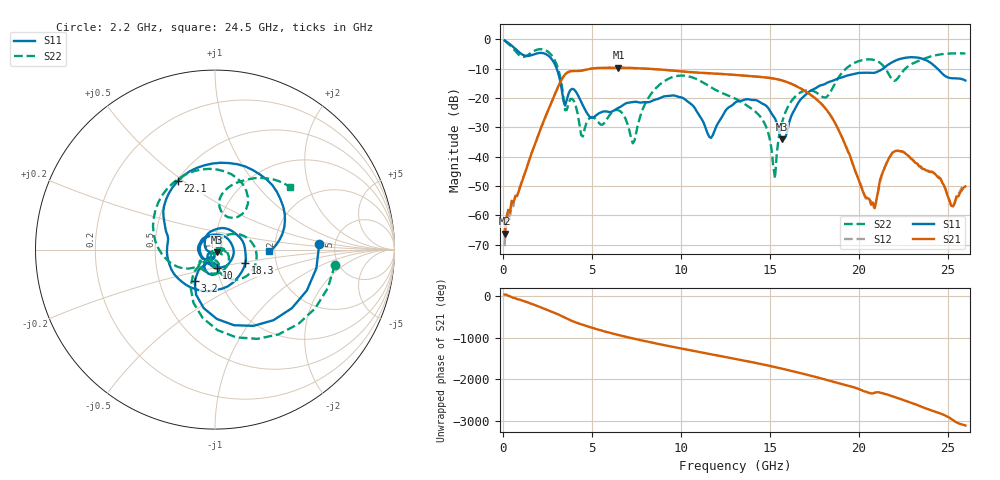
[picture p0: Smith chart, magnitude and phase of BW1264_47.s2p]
!Keysight Technologies,N5245B,MY57181159,A.13.60.06
!Date: Friday, December 18, 2020 23:54:32
!Correction: S11(Full 2 Port(1,2))
!S21(Full 2 Port(1,2))
!S12(Full 2 Port(1,2))
!S22(Full 2 Port(1,2))
!S2P File: Measurements: S11, S21, S12, S22:
# Hz S  dB  R 50
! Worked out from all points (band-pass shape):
!   260 points, 100 MHz to 26 GHz, reference 50 ohm
!   highest |S21| = -9.73 dB at 6.5 GHz (marker M1); lowest = -66.2 dB at 100 MHz (marker M2)
!   |S21| within 3 dB of the highest: 3.411 GHz to 14.2 GHz (10.79 GHz wide, 123 % of centre)
!   lowest |S11| = -34.1 dB at 15.7 GHz (marker M3), VSWR 1.04, Z = 51.2 - j1.63 ohm
!   |S11| at or under -10 dB: 3.025 GHz to 21.38 GHz (18.36 GHz wide, 150 % of centre); 24.42 GHz to end of sweep
!   |S22| runs from -47.5 to -0.5 dB; largest |S21 - S12| = 0.00049
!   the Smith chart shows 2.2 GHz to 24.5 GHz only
!   S11 on the Smith chart (normalised r, x): 2.2 GHz: 3.74, +0.38; 3.2 GHz: 0.75, -0.28; 10 GHz: 1.00, -0.21; 18.3 GHz: 1.39, -0.21; 22.1 GHz: 0.51, +0.48; 24.5 GHz: 1.85, -0.04
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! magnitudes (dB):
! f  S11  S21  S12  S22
! 100 MHz  -0.4  -66.2  -70.5  -0.5
! 300 MHz  -1.3  -58.2  -58.2  -1.5
! 2.2 GHz  -4.7  -29.4  -29.4  -3.4
! 3.2 GHz  -13.6  -15.0  -15.0  -12.1
! 4.5 GHz  -22.6  -10.6  -10.6  -33.1
! 6.5 GHz  -23.4  -9.7  -9.7  -24.2
! 7.3 GHz  -21.5  -9.8  -9.8  -35.5
! 8.8 GHz  -20.2  -10.3  -10.3  -15.6
! 10 GHz  -19.8  -11.0  -11.0  -12.4
! 11.7 GHz  -33.7  -11.7  -11.7  -16.4
! 13.1 GHz  -21.4  -12.2  -12.2  -20.3
! 14.7 GHz  -22.3  -13.0  -13.0  -28.6
! 15.3 GHz  -27.1  -13.5  -13.5  -47.5
! 15.7 GHz  -34.1  -14.1  -14.1  -28.2
! 17.4 GHz  -17.2  -19.4  -19.4  -17.6
! 18.3 GHz  -14.7  -24.9  -24.9  -19.0
! 20.9 GHz  -11.4  -57.6  -58.0  -7.1
! 21.7 GHz  -8.5  -40.6  -40.6  -12.0
! 22.1 GHz  -7.2  -38.0  -38.1  -14.0
! 24.5 GHz  -10.5  -47.3  -46.8  -5.3
! 25.3 GHz  -13.3  -57.0  -57.5  -4.9
! 26 GHz  -14.1  -50.2  -50.2  -4.9
